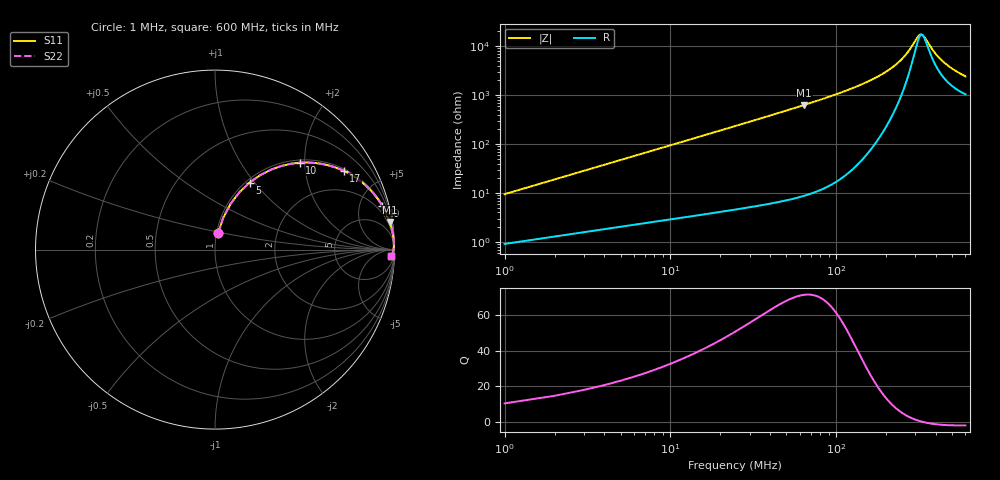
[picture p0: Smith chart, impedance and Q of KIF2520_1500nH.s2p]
!version-2
!date-12.2020
!Series
# MHz S RI R 50
!Freq ReS11 ImS11 ReS21 ImS21 ReS12 ImS12 ReS22 ImS22
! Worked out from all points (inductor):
!   600 points, 1 MHz to 600 MHz, reference 50 ohm
!   read as one part in series: L = 1.5 uH near 4 MHz
!   highest Q = 71.6 at 64 MHz (marker M1), where L = 1.56 uH
!   self-resonance near 328.9 MHz
!   S11 on the Smith chart (normalised r, x): 1 MHz: 1.02, +0.19; 5 MHz: 1.04, +0.94; 10 MHz: 1.06, +1.89; 17 MHz: 1.08, +3.21; 40 MHz: 1.12, +7.66; 600 MHz: 22, -44
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1  0.0176 0.0918  0.9824 -0.0918  0.9824 -0.0918  0.0176 0.0918
3  0.0863 0.2543  0.9137 -0.2543  0.9137 -0.2543  0.0863 0.2543
5  0.1923 0.3731  0.8077 -0.3731  0.8077 -0.3731  0.1923 0.3731
7  0.3101 0.4446  0.6899 -0.4446  0.6899 -0.4446  0.3101 0.4446
10  0.472 0.4842  0.528 -0.4842  0.528 -0.4842  0.472 0.4842
13  0.5985 0.4769  0.4015 -0.4769  0.4015 -0.4769  0.5985 0.4769
17  0.7163 0.4392  0.2837 -0.4392  0.2837 -0.4392  0.7163 0.4392
21  0.7931 0.3946  0.2069 -0.3946  0.2069 -0.3946  0.7931 0.3946
26  0.8541 0.3435  0.1459 -0.3435  0.1459 -0.3435  0.8541 0.3435
40  0.9328 0.2426  0.0672 -0.2426  0.0672 -0.2426  0.9328 0.2426
64  0.9732 0.1547  0.0268 -0.1547  0.0268 -0.1547  0.9732 0.1547
101  0.9896 0.0937  0.0104 -0.0937  0.0104 -0.0937  0.9896 0.0937
201  0.9964 0.0325  0.00358 -0.0325  0.00358 -0.0325  0.9964 0.0325
255  0.996 0.0162  0.00396 -0.0162  0.00396 -0.0162  0.996 0.0162
301  0.995 0.00552  0.00499 -0.00552  0.00499 -0.00552  0.995 0.00552
317  0.9945 0.00228  0.00545 -0.00228  0.00545 -0.00228  0.9945 0.00228
330  0.9941 -0.000215  0.00586 0.000215  0.00586 0.000215  0.9941 -0.000215
376  0.9925 -0.00821  0.00752 0.00821  0.00752 0.00821  0.9925 -0.00821
401  0.9915 -0.0121  0.00854 0.0121  0.00854 0.0121  0.9915 -0.0121
445  0.9895 -0.0184  0.0105 0.0184  0.0105 0.0184  0.9895 -0.0184
501  0.9867 -0.0254  0.0133 0.0254  0.0133 0.0254  0.9867 -0.0254
600  0.9812 -0.036  0.0188 0.036  0.0188 0.036  0.9812 -0.036
